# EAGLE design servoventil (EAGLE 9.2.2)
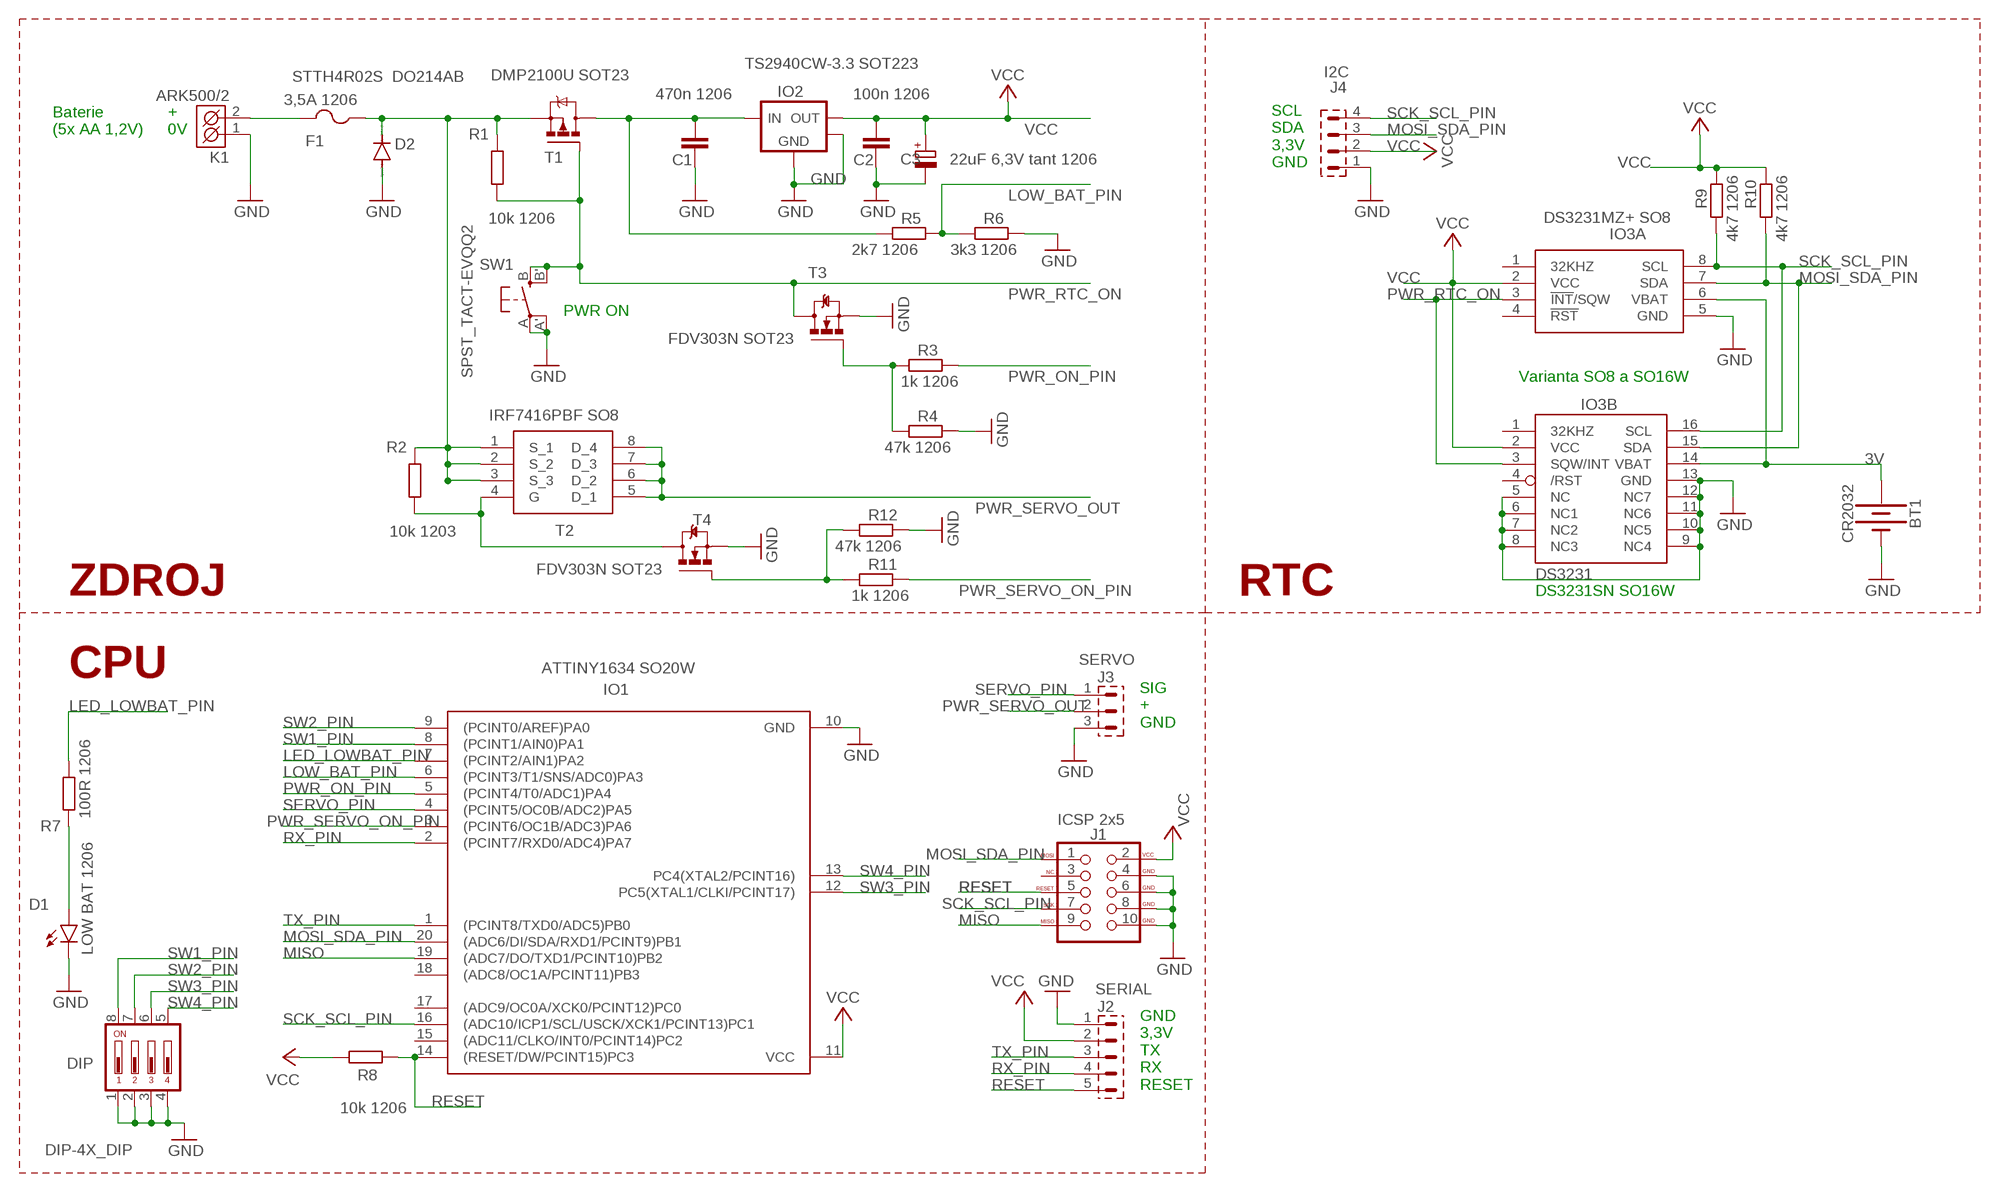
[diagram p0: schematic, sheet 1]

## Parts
BT1  CR2032  BATTERY-20MM_PTH  [BATTCOM_20MM_PTH]
C1  470n 1206  C-EUC1206  [C1206]
C2  100n 1206  C-EUC1206  [C1206]
C3  22uF 6,3V tant 1206  CPOL-EUCT3216  [CT3216]
D1  LOW BAT 1206  LED1206  [LED-1206]
D2  STTH4R02S DO214AB  DIODE-DO214AA  [DO214AA]
DIP  DIP-4X_DIP  [DIP-4X]
F1  3,5A 1206  PTCFUSE-1206  [R1206]
IO1  ATTINY1634 SO20W  ATTINY1634-SU  [SOIC20]
IO2  TS2940CW-3.3 SOT223  MCP1825_SOT223  [SOT-223-3]
IO3A  DS3231MZ+ SO8  DS3231MZ+  [SOIC127P600X175-8N]
IO3B  DS3231SN SO16W  DS3231/SO  [SO16W]
J1  ICSP 2x5  AVR_SPI_PROG_5X2LOCK  [2X5-SHROUDED_LOCK]
J2  SERIAL  S1G5_JUMP  [S1G5_JUM]
J3  SERVO  S1G3_JUMP  [S1G3_JUM]
J4  I2C  S1G4_JUMP  [S1G4_JUM]
K1  ARK500/2  [ARK500/2]
R1  10k 1206  R-EU_R1206  [R1206]
R2  10k 1203  R-EU_R1206  [R1206]
R3  1k 1206  R-EU_R1206  [R1206]
R4  47k 1206  R-EU_R1206  [R1206]
R5  2k7 1206  R-EU_R1206  [R1206]
R6  3k3 1206  R-EU_R1206  [R1206]
R7  100R 1206  R-EU_R1206  [R1206]
R8  10k 1206  R-EU_R1206  [R1206]
R9  4k7 1206  R-EU_R1206  [R1206]
R10  4k7 1206  R-EU_R1206  [R1206]
R11  1k 1206  R-EU_R1206  [R1206]
R12  47k 1206  R-EU_R1206  [R1206]
SW1  SPST_TACT-EVQQ2  [EVQ-Q2]
T1  DMP2100U SOT23  MOSFET-P-SOT23  [SOT-23]
T2  IRF7416PBF SO8  IRF7416PBF  [SOIC127P600X175-8N]
T3  FDV303N SOT23  MOSFET-N-SOT23  [SOT-23]
T4  FDV303N SOT23  MOSFET-N-SOT23  [SOT-23]

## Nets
3V: BT1.1(+) IO3A.6(VBAT) IO3B.14(VBAT)
6V: C1.1 IO2.1(VIN) R5.2 T1.3(D)
GND: BT1.2(-) C1.2 C2.2 C3.- D1.C D2.A DIP.1 DIP.2 DIP.3 DIP.4 IO1.10(GND) IO2.2(GND) IO2.4(HEATSINK) IO3A.5(GND) IO3B.5(NC) IO3B.6(NC1) IO3B.7(NC2) IO3B.8(NC3) IO3B.9(NC4) IO3B.10(NC5) IO3B.11(NC6) IO3B.12(NC7) IO3B.13(GND) J1.4(GND) J1.6(GND) J1.8(GND) J1.10(GND) J2.1 J3.3 J4.1 K1.1(K1) R4.1 R6.1 R12.1 SW1.A'(P1) SW1.A(P) T3.2(S) T4.2(S)
LED_LOWBAT_PIN: IO1.7((PCINT2/AIN1)PA2) R7.1
LOW_BAT_PIN: IO1.6((PCINT3/T1/SNS/ADC0)PA3) R5.1 R6.2
MISO: IO1.19((ADC7/DO/TXD1/PCINT10)PB2) J1.9(MISO)
MOSI_SDA_PIN: IO1.20((ADC6/DI/SDA/RXD1/PCINT9)PB1) IO3A.7(SDA) IO3B.15(SDA) J1.1(MOSI) J4.3 R10.2
N$1: F1.2 K1.2(K2)
N$2: D2.C F1.1 R1.2 R2.2 T1.2(S) T2.1(S_1) T2.2(S_2) T2.3(S_3)
N$3: R3.2 R4.2 T3.1(G)
N$4: R2.1 T2.4(G) T4.3(D)
N$5: R11.2 R12.2 T4.1(G)
N$12: D1.A R7.2
PWR_ON_PIN: IO1.5((PCINT4/T0/ADC1)PA4) R3.1
PWR_RTC_ON: IO3A.3(!INT!/SQW) IO3B.3(SQW/INT) R1.1 SW1.B'(S1) SW1.B(S) T1.1(G) T3.3(D)
PWR_SERVO_ON_PIN: IO1.3((PCINT6/OC1B/ADC3)PA6) R11.1
PWR_SERVO_OUT: J3.2 T2.5(D_1) T2.6(D_2) T2.7(D_3) T2.8(D_4)
RESET: IO1.14((RESET/DW/PCINT15)PC3) J1.5(RESET) J2.5 R8.2
RX_PIN: IO1.2((PCINT7/RXD0/ADC4)PA7) J2.4
SCK_SCL_PIN: IO1.16((ADC10/ICP1/SCL/USCK/XCK1/PCINT13)PC1) IO3A.8(SCL) IO3B.16(SCL) J1.7(SCK) J4.4 R9.2
SERVO_PIN: IO1.4((PCINT5/OC0B/ADC2)PA5) J3.1
SW1_PIN: DIP.8 IO1.8((PCINT1/AIN0)PA1)
SW2_PIN: DIP.7 IO1.9((PCINT0/AREF)PA0)
SW3_PIN: DIP.6 IO1.12(PC5(XTAL1/CLKI/PCINT17))
SW4_PIN: DIP.5 IO1.13(PC4(XTAL2/PCINT16))
TX_PIN: IO1.1((PCINT8/TXD0/ADC5)PB0) J2.3
VCC: C2.1 C3.+ IO1.11(VCC) IO2.3(VOUT) IO3A.2(VCC) IO3B.2(VCC) J1.2(VCC) J2.2 J4.2 R8.1 R9.1 R10.1
Unconnected: IO1.15((ADC11/CLKO/INT0/PCINT14)PC2) IO1.17((ADC9/OC0A/XCK0/PCINT12)PC0) IO1.18((ADC8/OC1A/PCINT11)PB3) IO3A.1(32KHZ) IO3A.4(!RST) IO3B.1(32KHZ) IO3B.4(/RST) J1.3(NC)

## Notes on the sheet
- Baterie 
  (5x AA 1,2V)
- +
  0V
- SCL
  SDA
  3,3V
  GND
- PWR ON
- Varianta SO8 a SO16W
- ZDROJ | RTC | DS3231SN SO16W
- CPU
- SIG
  +
  GND
- GND
  3,3V
  TX
  RX
  RESET

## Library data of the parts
BT1 = SparkFun-Batteries:BATTERY: Battery - Single Cell; PROD_ID: BATT-09031; SF_SKU: PRT-00783
C1 C2 = rcl:C-EU: CAPACITOR, European symbol; SPICEPREFIX: C
C3 = rcl:CPOL-EU: POLARIZED CAPACITOR, European symbol; SPICEPREFIX: C
D1 = SparkFun-LED:LED: LED (Generic)
D2 = diode:DIODE-: DIODE
DIP = #PaJa_prepinace:DIP-4X: DIP Prepinac - 4x
F1 = adafruit:PTCFUSE: PTC fuses, resettable thermistors
IO1 = bt_avr:ATTINY1634: ATtiny1634 ATtiny1634 is a low-power CMOS 8-bit microcontrollers based on the AVR enhanced RISC architecture. By executing powerful instructions in a single clock cycle, the ATtiny1634 achieves throughputs approaching 1 MIPS per MHz allowing the system designer to optimize power consumption versus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
IO2 = bt_regulator:MCP1825: Microchip MCP1824 LDO Voltage Regulator The MCP1825/MCP1825S is a 500 mA Low Dropout (LDO) linear regulator that provides high current and low output voltages. Datasheet.pdf
IO3A = SamacSys_Parts:DS3231MZ+: Real Time Clock 5+/-ppm RTC Source: Datasheet; DESCRIPTION: Real Time Clock 5+/-ppm RTC; HEIGHT: 1.75mm; MANUFACTURER_NAME: Maxim Integrated; MANUFACTURER_PART_NUMBER: DS3231MZ+; MOUSER_PART_NUMBER: 700-DS3231MZ+
IO3B = adafruit:DS3231
J1 = SparkFun-Connectors:AVR_SPI_PROG_5X2: AVR 10-pin ICSP Header This is the standard AVR In Circuit Serial Programming header. Minimal, but includes pin one indicator. Works with standard Olimex programmers. SparkFun Products: 2x5 AVR ICSP Male Header - PTH 2x5 Pin Shrouded Header - PTH2; PROD_ID: CONN-08671; SF_ID: PRT-08506
J2 = #PaJa_konektory:S1G5_JUMP: Radove konektory - koliky - 5x
J3 = #PaJa_konektory:S1G3_JUMP: Radove konektory - koliky - 3x
J4 = #PaJa_konektory:S1G4_JUMP: Radove konektory - koliky - 4x
K1 = #PaJa_konektory:ARK500/2: Svorkovnice - roztec 5mm - dvojita
R1-R12 = rcl:R-EU_: RESISTOR, European symbol; SPICEPREFIX: R
SW1 = adafruit:SPST_TACT: SMT 6mm switch, EVQQ2 series http://www.ladyada.net/library/eagle
T1 = bt_transistor:MOSFET-P: P-Channel MOSFET with integrated body diode
T2 = SamacSys_Parts:IRF7416PBF: MOSFET P-Channel 30V 10A HEXFET SOIC8 Infineon IRF7416PBF P-channel MOSFET Transistor, 10 A, 30 V, 8-Pin SOIC Source: Datasheet; DESCRIPTION: MOSFET P-Channel 30V 10A HEXFET SOIC8 Infineon IRF7416PBF P-channel MOSFET Transistor, 10 A, 30 V, 8-Pin SOIC; HEIGHT: 1.75mm; MANUFACTURER_NAME: Infineon; MANUFACTURER_PART_NUMBER: IRF7416PBF; MOUSER_PART_NUMBER: 942-IRF7416PBF
T3 T4 = bt_transistor:MOSFET-N: N-Channel MOSFET

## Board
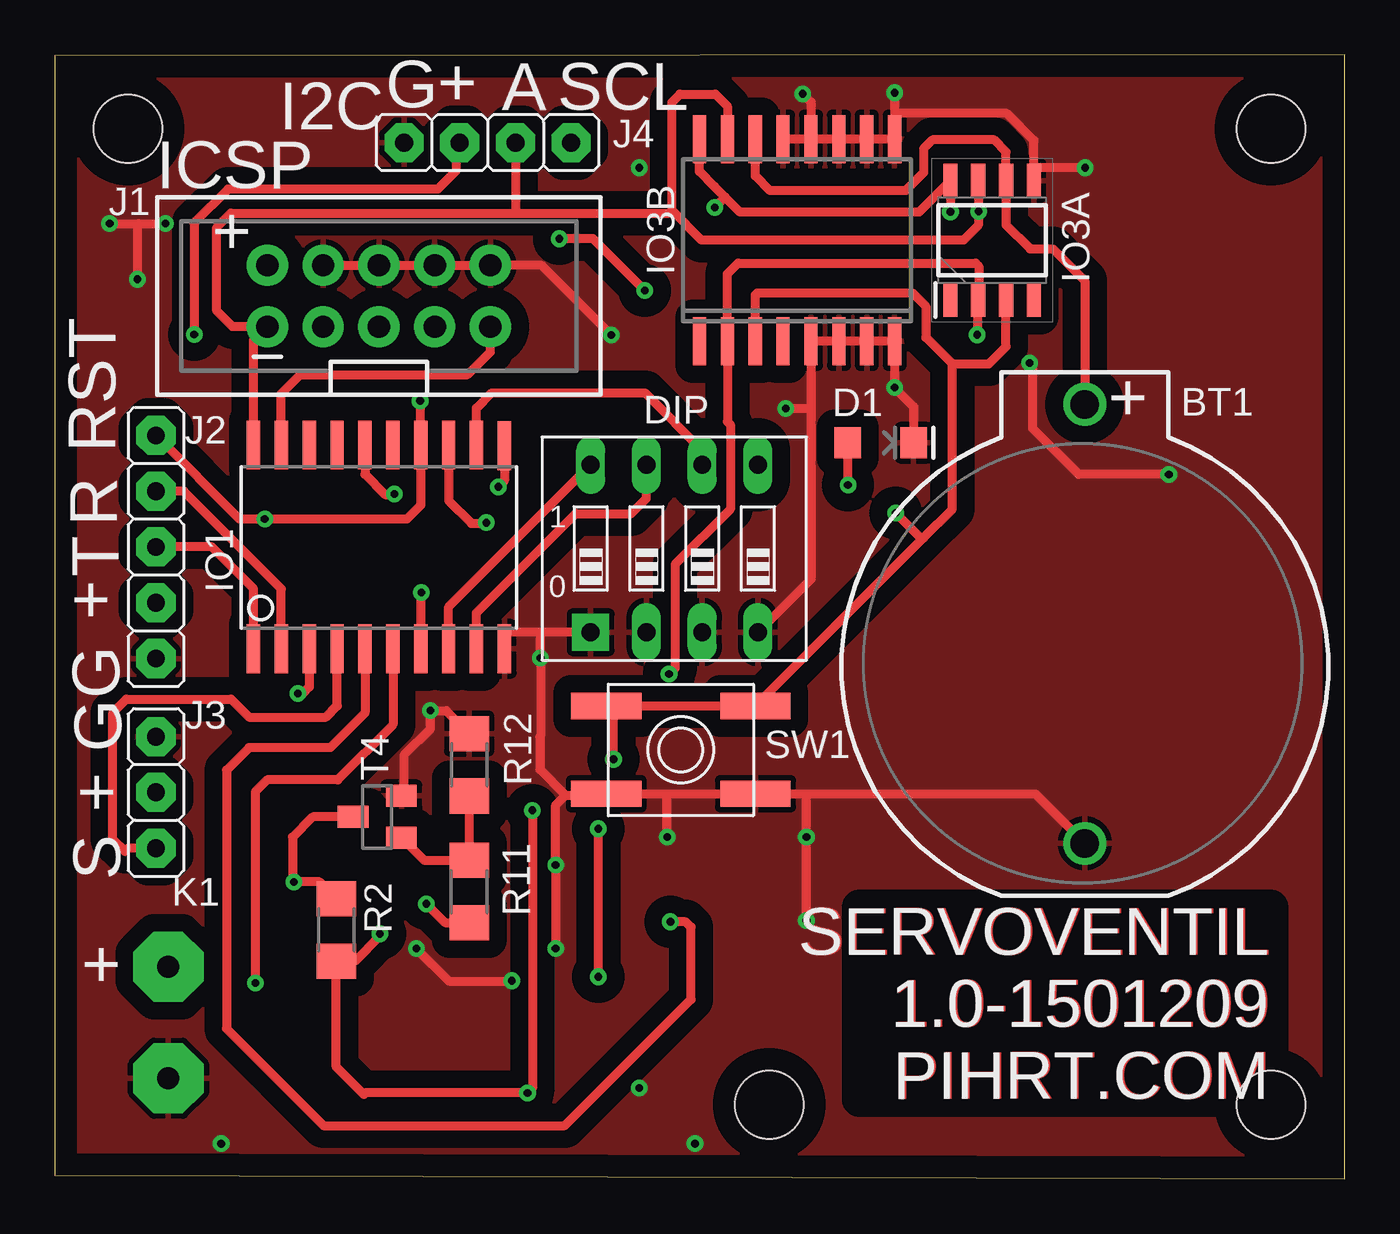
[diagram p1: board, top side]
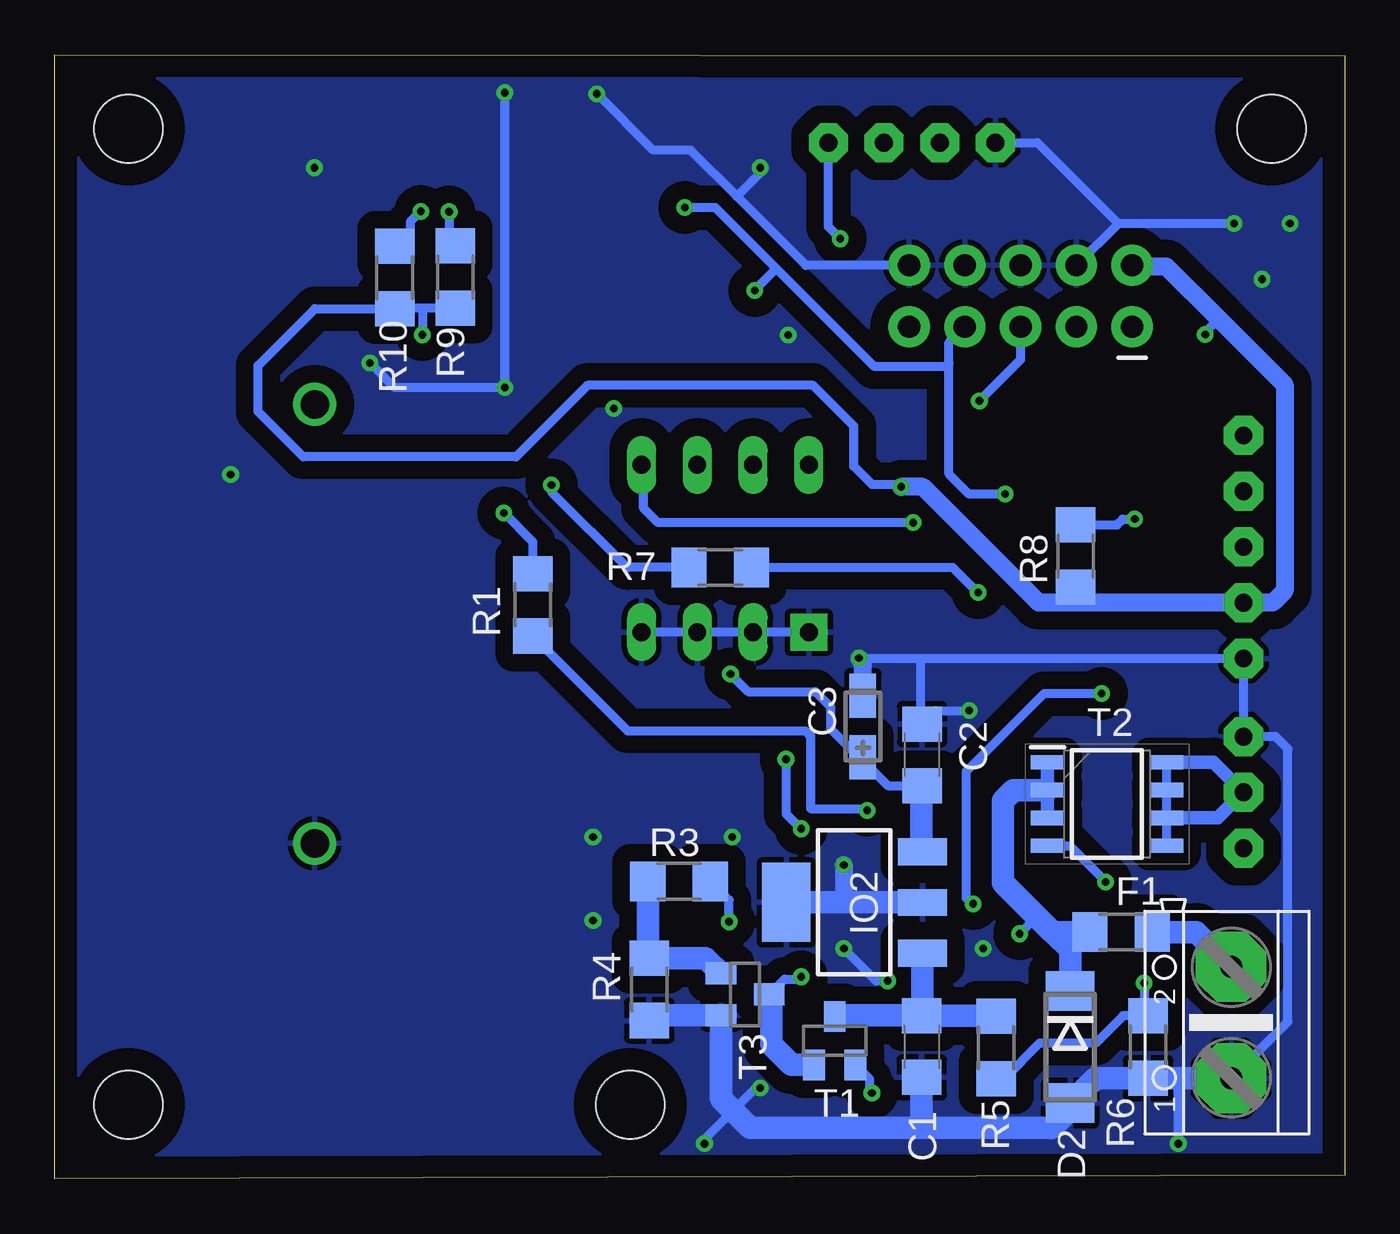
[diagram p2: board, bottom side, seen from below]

Size 58.76 x 51.19 mm. Coordinates in mm from the lower left corner, seen from the top.
Outline: 0,0.15 58.76,0 58.76,51.19 0,51.16 0,0.15
Copper layers (1*16): Top 0.035mm / dielectric 1.5mm / Bottom 0.035mm
Design rules "default": minimum track width 6mil, minimum drill 0.35mm, track to track 6mil, track to pad 6mil, pad to pad 6mil, via to via 6mil, smd to smd 6mil, copper to edge 40mil, drill to drill 6mil, minimum pad ring 10mil, minimum via ring 8mil, stop-mask expansion 4mil, vias tented up to drill 0mil, thermal gap 10mil
Holes 3.1 mm at 3.34,47.83 55.41,47.83 55.41,3.38 32.55,3.38

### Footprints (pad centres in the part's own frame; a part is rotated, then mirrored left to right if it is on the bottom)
BATTCOM_20MM_PTH = drill 1.3: 1 11.85,0; 2 -8.15,0
C1206 = smd 1.6 x 1.8: 1 -1.4,0; 2 1.4,0
CT3216 = smd 2 x 1.2: + -1.4,0; - 1.4,0
LED-1206 = smd 1.2 x 1.4: A -1.5,0; C 1.5,0
DO214AA = smd 1.8 x 2.2: A 2.55,0; C -2.55,0
DIP-4X = drill 0.813 pad 1.676 square: 1 -3.81,-3.81 | drill 0.813 pad 1.27 long: 2 -1.27,-3.81; 3 1.27,-3.81; 4 3.81,-3.81; 5 3.81,3.81; 6 1.27,3.81; 7 -1.27,3.81; 8 -3.81,3.81
R1206 = smd 1.6 x 1.803: 1 -1.422,0; 2 1.422,0
SOIC20 = smd 0.61 x 2.21: 1 -5.715,-4.636; 2 -4.445,-4.636; 3 -3.175,-4.636; 4 -1.905,-4.636; 5 -0.635,-4.636; 6 0.635,-4.636; 7 1.905,-4.636; 8 3.175,-4.636; 9 4.445,-4.636; 10 5.715,-4.636; 11 5.715,4.61; 12 4.445,4.636; 13 3.175,4.636; 14 1.905,4.636; 15 0.635,4.636; 16 -0.635,4.636; 17 -1.905,4.636; 18 -3.175,4.636; 19 -4.445,4.636; 20 -5.715,4.636
SOT-223-3 = smd 1.219 x 2.235: 1 -2.311,-3.099; 2 0,-3.099; 3 2.311,-3.099 | smd 3.6 x 2.2: 4 0,3.099
SOIC127P600X175-8N = smd 1.525 x 0.65: 1 -2.712,1.905; 2 -2.712,0.635; 3 -2.712,-0.635; 4 -2.712,-1.905; 5 2.712,-1.905; 6 2.712,-0.635; 7 2.712,0.635; 8 2.712,1.905
SO16W = smd 0.6 x 2.2: 1 -4.445,-4.6; 2 -3.175,-4.6; 3 -1.905,-4.6; 4 -0.635,-4.6; 5 0.635,-4.6; 6 1.905,-4.6; 7 3.175,-4.6; 8 4.445,-4.6; 9 4.445,4.6; 10 3.175,4.6; 11 1.905,4.6; 12 0.635,4.6; 13 -0.635,4.6; 14 -1.905,4.6; 15 -3.175,4.6; 16 -4.445,4.6
2X5-SHROUDED_LOCK = drill 1.016 pad 1.88: 1 -1.397,5.08; 2 1.397,5.08; 3 -1.397,2.54; 4 1.397,2.54; 5 -1.397,0; 6 1.397,0; 7 -1.397,-2.54; 8 1.397,-2.54; 9 -1.397,-5.08; 10 1.397,-5.08
S1G5_JUM = drill 0.813 pad 1.778 octagon: 1 -5.08,0; 2 -2.54,0; 3 0,0; 4 2.54,0; 5 5.08,0
S1G3_JUM = drill 0.813 pad 1.778 octagon: 1 -2.54,0; 2 0,0; 3 2.54,0
S1G4_JUM = drill 0.813 pad 1.778 octagon: 1 -3.81,0; 2 -1.27,0; 3 1.27,0; 4 3.81,0
ARK500/2 = drill 1 pad 3.2 octagon: 1 -2.54,0; 2 2.54,0
EVQ-Q2 = smd 3.2 x 1.2: A -3.4,-2; A' 3.4,-2; B -3.4,2; B' 3.4,2
SOT-23 = smd 1 x 1.4: 1 -0.95,-1.1; 2 0.95,-1.1; 3 0,1.1

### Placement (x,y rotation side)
BT1  46.93,23.42 90 top
C1  19.27,6.02 270 bottom
C2  19.25,19.3 90 bottom
C3  21.95,20.6 90 bottom
D1  37.62,33.52 0 top
D2  12.5,6 270 bottom
DIP  28.22,28.71 0 top
F1  10.18,11.24 0 bottom
IO1  14.77,28.78 0 top
IO2  22.34,12.59 90 bottom
IO3A  42.71,42.75 90 top
IO3B  33.82,42.75 0 top
J1  14.77,40.21 90 top
J2  4.61,28.78 90 top
J3  4.61,17.6 90 top
J4  19.71,47.19 0 top
K1  5.17,7.12 90 bottom
R1  36.99,26.14 270 bottom
R2  12.82,11.33 270 top
R3  30.33,13.55 180 bottom
R4  31.68,8.63 90 bottom
R5  15.87,5.98 90 bottom
R6  8.96,6.01 90 bottom
R7  28.46,27.84 180 bottom
R8  12.26,28.36 90 bottom
R9  40.52,41.07 90 bottom
R10  43.28,41.05 90 bottom
R11  18.88,13.09 90 top
R12  18.88,18.86 270 top
SW1  28.52,19.53 0 top
T1  23.23,6.29 0 bottom
T2  10.83,17.07 0 bottom
T3  27.31,8.4 270 bottom
T4  14.69,16.49 90 top

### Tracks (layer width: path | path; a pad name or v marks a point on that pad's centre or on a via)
3V
  Top 0.406: IO3B.14 31.91,45.68 32.59,45.01 38.75,45.01 39.58,45.83 39.58,46.9 39.99,47.32 42.8,47.32 43.34,46.77 IO3A.6 43.34,43.45 44.44,42.35 45.47,42.35 46.93,40.89 BT1.1
6V
  Bottom 1.016: IO2.1 19.24,7.45 | 19.24,7.45 C1.1 15.89,7.42 R5.2 | T1.3 23.17,7.45 19.24,7.45
GND  (via drill 0.35)
  Top 0.406: DIP.1 22.27,24.9 | 22.27,24.9 20.44,24.9 20.44,24.89 20.48,24.84 IO1.10 | J1.4 J1.6 J1.8 J1.10 22.18,41.6 v25.36,38.43 | 34.45,35.09 IO3B.5 IO3B.6 IO3B.7 IO3B.8 38.26,36.24 v38.26,36.03 39.12,35.17 D1.C | 34.45,35.09 34.45,27.31 DIP.4 | IO3B.9 IO3B.10 IO3B.11 IO3B.12 | IO3B.12 IO3B.13 | v38.26,49.47 38.26,48.53 | 38.26,48.53 IO3B.9 | IO3B.9 | IO3A.5 44.61,46 | 44.61,46 44.61,47.28 43.37,48.53 38.26,48.53 | v34.07,49.42 34.45,49.04 IO3B.12 | 22.27,24.9 22.12,24.75 v22.12,23.72 22.12,20.15 22.1,20.12 22.1,18.64 23.27,17.47 | 27.92,17.53 SW1.A 25.06,17.47 23.27,17.47 | 27.92,17.53 SW1.A' 34.28,17.53 | 34.28,17.53 44.67,17.53 BT1.2 | T4.2 15.92,17.56 15.92,19.31 17.11,20.5 v17.11,21.32 17.83,21.32 R12.1 | v22.82,10.49 v22.82,14.3 22.82,17.01 23.27,17.47 | v34.25,11.76 v34.25,15.57 34.25,17.5 34.28,17.53 | v50.76,32.08 46.65,32.08 44.56,34.17 44.56,37 v44.41,37.16 | v33.3,35.09 34.45,35.09 | v2.5,43.51 3.82,43.51 | 3.82,43.51 v5.04,43.51 | v3.77,40.97 3.77,43.45 3.82,43.51 | v46.95,46.05 44.66,46.05 44.61,46 | v27.9,15.57 27.9,17.51 27.92,17.53 | v16.47,10.49 17.95,9 20.74,9 20.76,9.02 v20.82,9.02
  Bottom 0.406: v38.26,49.47 v38.26,36.03 43.28,36.03 v44.41,37.16 | J1.10 24.55,41.6 27.69,44.75 | 27.69,44.75 29.79,46.85 31.5,46.85 v34.07,49.42 | J3.3 J2.1 19.31,23.7 | J3.3 | 19.31,23.7 22.11,23.7 22.12,23.68 | 22.16,23.65 22.12,23.68 | 22.12,23.68 v22.12,23.72 | K1.1 2.59,7.16 2.59,19.58 3.15,20.14 J3.3 | 19.31,23.7 19.31,20.76 C2.2 18.63,21.32 v17.11,21.32 | DIP.1 DIP.2 DIP.3 DIP.4 | v5.04,43.51 10.32,43.51 | 10.32,43.51 J1.4 | v29.17,1.6 29.17,1.79 27.86,3.1 26.82,4.14 v26.63,4.14 | v26.63,46.05 26.63,45.82 27.69,44.75 | v7.58,1.6 7.58,4.52 7.63,4.58 | v20.82,9.02 21.34,9.02 v22.82,10.49 | J4.1 14,47.19 10.32,43.51
  Bottom 0.813: v22.82,14.3 22.82,12.62 22.84,12.59 | C3.- 21.95,23.54 22.11,23.7
  Bottom 1.016: K1.1 7.63,4.58 8.94,4.58 R6.1 11.37,4.59 D2.A 12.5,3.16 13.37,2.3 13.39,2.32 18.89,2.32 | C1.2 19.27,2.71 18.89,2.32 | R4.1 31.44,7.45 T3.2 28.41,3.65 27.86,3.1 27.09,2.32 18.89,2.32 | IO2.2 22.84,12.59 IO2.4
  pour Bottom (isolate 0.813): -0.47,51.64 59.22,51.64 59.22,-0.43 -0.47,-0.43
  pour Top (isolate 0.813): -0.47,51.64 59.22,51.64 59.22,-0.43 -0.47,-0.43
LED_LOWBAT_PIN  (via drill 0.35)
  Top 0.406: v16.69,26.7 16.67,26.68 IO1.7
  Bottom 0.406: R7.1 17.86,27.84 16.78,26.76 16.72,26.76 16.72,26.73 v16.69,26.7
LOW_BAT_PIN  (via drill 0.35)
  Top 0.406: v9.13,8.92 v9.13,8.93 9.13,17.62 9.68,18.17 12.89,18.17 15.4,20.68 IO1.6
  Bottom 0.406: R5.1 15.51,4.56 13.9,6.18 11.34,6.18 10.09,7.43 R6.2 9.13,7.61 v9.13,8.92
MISO
  Top 0.406: IO1.19 10.32,35.76 11.18,36.62 18.8,36.62 19.85,37.67 J1.9
MOSI_SDA_PIN  (via drill 0.35)
  Top 0.406: IO1.20 9.05,38.17 J1.1 8.09,38.81 7.37,39.53 7.37,43.34 8.02,43.98 21.05,43.98 | v42.09,44.06 42.07,44.08 42.07,44.17 IO3A.7 42.07,43.43 41.39,42.76 29.47,42.76 28.11,44.12 | 28.11,44.12 28.11,49.03 28.48,49.4 30.09,49.4 30.64,48.85 IO3B.15 | 21.05,43.98 27.97,43.98 28.11,44.12 | J4.3 20.98,44.04 21.05,43.98
  Bottom 0.406: v42.09,44.06 42.57,43.58 42.57,43.03 43.13,42.48 R10.2
N$1
  Bottom 1.016: F1.2 6.75,11.24 K1.2
N$2  (via drill 0.35)
  Top 0.406: v14.8,11.16 14.83,11.14 14.83,11.06 13.67,9.91 R2.2 12.82,5.1 14.08,3.85 14.14,3.91 v21.53,3.91 21.76,4.13 v21.76,16.78
  Bottom 0.406: v14.8,11.16 14.08,11.88 14.08,12 | T1.2 21.65,4.56 21.65,4.03 v21.53,3.91 | R1.2 32.66,20.4 24.57,20.4 24.34,20.16 24.34,16.86 21.83,16.86 v21.76,16.78 | 12.5,10.42 12.5,10.34
  Bottom 0.61: T2.1 T2.2 T2.3
  Bottom 1.016: 12.5,10.34 D2.C | T2.2 15.09,17.71 15.57,17.23 15.57,13.49 14.08,12 13.32,11.24 | 13.32,11.24 12.5,10.42 | F1.1 13.32,11.24
N$3
  Bottom 1.016: T3.1 29.11,10.05 R4.2 31.75,10.12 R3.2
N$4  (via drill 0.35)
  Top 0.406: R2.1 12.06,13.52 v10.88,13.52 10.83,13.57 10.83,15.56 11.75,16.49 T4.3
  Bottom 0.406: T2.4 12.53,15.17 v10.88,13.52
N$5
  Top 0.406: T4.1 16.82,14.51 R11.2 R12.2
N$12  (via drill 0.35)
  Top 0.406: v36.14,31.6 36.14,33.51 D1.A
  Bottom 0.406: R7.2 32.66,27.84 32.68,27.82 36.1,31.24 36.1,31.46 36.14,31.49 v36.14,31.6
PWR_ON_PIN  (via drill 0.35)
  Top 0.406: IO1.5 14.13,21.22 12.55,19.64 8.85,19.64 7.82,18.61 7.82,6.84 12.24,2.42 23.23,2.42 28.98,8.18 28.98,11.47 28.74,11.71 v28.05,11.71
  Bottom 0.406: v28.05,11.71 28.05,12.69 R3.1
PWR_RTC_ON  (via drill 0.35)
  Top 0.406: IO3B.3 31.91,40.26 32,40.35 39.07,40.35 39.68,39.73 39.68,38.32 40.89,37.12 | 40.89,37.12 42.55,37.12 43.34,37.9 IO3A.3 | SW1.B 25.44,21.53 | 25.44,21.53 SW1.B' 39.57,29.19 | 39.57,29.19 40.89,30.5 40.89,37.12 | v38.31,30.32 39.45,29.19 39.57,29.19 | v24.76,9.2 v24.76,15.94 | v25.45,19.11 25.45,21.52 25.44,21.53
  Bottom 0.406: R1.1 36.99,29 v38.31,30.32 | v38.31,30.32 | T3.3 25.52,9.09 24.94,9.09 24.83,9.2 v24.76,9.2 | v24.76,15.94 25.45,16.63 v25.45,19.1 v25.45,19.11
  Bottom 1.016: T3.3 26.12,8.31 26.12,6.11 25.19,5.19 T1.1
PWR_SERVO_ON_PIN  (via drill 0.35)
  Top 0.406: IO1.3 11.59,22.4 11.29,22.1 v11.08,22.1 | v16.92,12.52 17.78,11.67 R11.1
  Bottom 0.406: v11.08,22.1 13.7,22.1 17.25,18.55 17.25,12.79 16.98,12.52 v16.92,12.52
PWR_SERVO_OUT
  Bottom 0.406: T2.8 T2.7 T2.6 T2.5
  Bottom 0.61: T2.8 5.98,18.98 J3.2 5.77,16.44 T2.6
RESET  (via drill 0.35)
  Top 0.406: J2.5 8.42,30.05 v9.56,30.05 16.04,30.05 16.67,30.68 IO1.14 16.67,35.4 v16.64,35.43
  Bottom 0.406: v16.64,35.43 14.77,37.31 J1.5 | R8.2 10.37,29.78 10.11,30.05 v9.56,30.05
RX_PIN
  Top 0.406: IO1.2 10.32,26.87 5.88,31.32 J2.4
SCK_SCL_PIN  (via drill 0.35)
  Top 0.406: IO1.16 14.13,32.09 15.05,31.16 15.45,31.16 v15.47,31.18 | v40.8,44.05 40.78,44.06 40.78,44.13 40.8,44.15 IO3A.8 39.37,44.03 31.22,44.03 30.54,44.71 | IO3B.16 29.37,45.88 30.06,45.19 30.54,44.71 | v30.06,44.24 30.54,44.71 | v26.88,40.45 24.52,42.82 v22.98,42.82
  Bottom 0.406: v15.47,31.18 17.12,31.18 18.02,32.09 18.02,37.16 | 18.02,37.16 18.02,38.09 J1.7 | v40.8,44.05 40.8,42.78 R9.2 | 18.02,37.16 18.2,36.98 21.42,36.98 25.93,41.5 | 25.93,41.5 28.67,44.24 v30.06,44.24 | 25.93,41.5 25.93,41.42 26.88,40.48 v26.88,40.45 | v22.98,42.82 23.52,43.36 J4.4
SERVO_PIN
  Top 0.406: J3.1 3.35,15.06 3.2,14.91 2.64,15.47 2.64,21.23 3.25,21.84 8.03,21.84 8.85,21.03 12.35,21.03 12.86,21.54 IO1.4
SW1_PIN
  Top 0.406: IO1.8 17.94,26.04 DIP.8
SW2_PIN
  Top 0.406: IO1.9 19.21,25.78 23.73,30.3 26.26,30.3 26.95,30.99 DIP.7
SW3_PIN
  Top 0.406: IO1.12 19.21,35.11 19.9,35.8 26.88,35.8 29.59,33.09 29.49,33 DIP.6
SW4_PIN  (via drill 0.35)
  Top 0.406: IO1.13 17.94,30.89 18.98,29.85 19.63,29.85 v19.66,29.88
  Bottom 0.406: v19.66,29.88 31.28,29.88 31.93,30.54 31.93,32.42 DIP.5
TX_PIN
  Top 0.406: IO1.1 9.05,26.87 7.15,28.78 J2.3
VCC  (via drill 0.35)
  Top 0.406: IO1.11 20.48,31.8 v20.2,31.52 | J4.2 18.27,47.01 18.27,45.91 17.44,45.08 7.89,45.08 6.35,43.54 v6.35,38.45 | v42.02,38.44 42.04,38.46 42.04,40 IO3A.2 42.09,40.06 42.09,41.56 41.94,41.71 31.13,41.71 30.64,41.22 IO3B.2 30.64,34.49 30.78,34.35 30.78,30.5 28.27,27.98 28.27,23.27 v27.98,22.99
  Bottom 0.406: v6.35,38.45 6.35,38.55 5.74,39.16 | R9.1 42.02,39.65 | 42.02,39.65 43.26,39.65 R10.1 46.92,39.63 49.51,37.04 49.51,34.94 47.45,32.88 37.76,32.88 34.49,36.14 24.21,36.14 22.36,34.28 22.36,32.45 21.52,31.61 20.29,31.61 v20.2,31.52 | v27.98,22.99 27.18,22.19 24.11,22.19 23.42,21.49 23.42,20.5 22.17,19.25 20.82,17.91 C2.1 | 42.02,39.65 v42.02,38.45 v42.02,38.44
  Bottom 0.813: J1.2 9.64,41.56 8.14,41.56 5.74,39.16 2.73,36.15 2.73,26.79 3.28,26.24 J2.2 12.21,26.24 | 12.21,26.24 13.94,26.24 19.22,31.52 v20.2,31.52 | R8.1 12.21,26.88 12.21,26.24 | C3.+ 22,19.25 22.17,19.25
  Bottom 1.016: IO2.3 19.28,14.94 19.28,17.87 C2.1

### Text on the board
Top: SERVOVENTIL / 1.0-1501209 / PIHRT.COM
tNames: G | + | I2C | A | SCL | ICSP | + | + | RST | R | T | + | G | G | + | S | + | SERVOVENTIL / 1.0-1501209 / PIHRT.COM

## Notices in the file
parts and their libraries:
SparkFun-LED: Licensing: Creative Commons ShareAlike 4.0 International - https://creativecommons.org/licenses/by-sa/4.0
Copyright (C) PaJa 2011-2014
